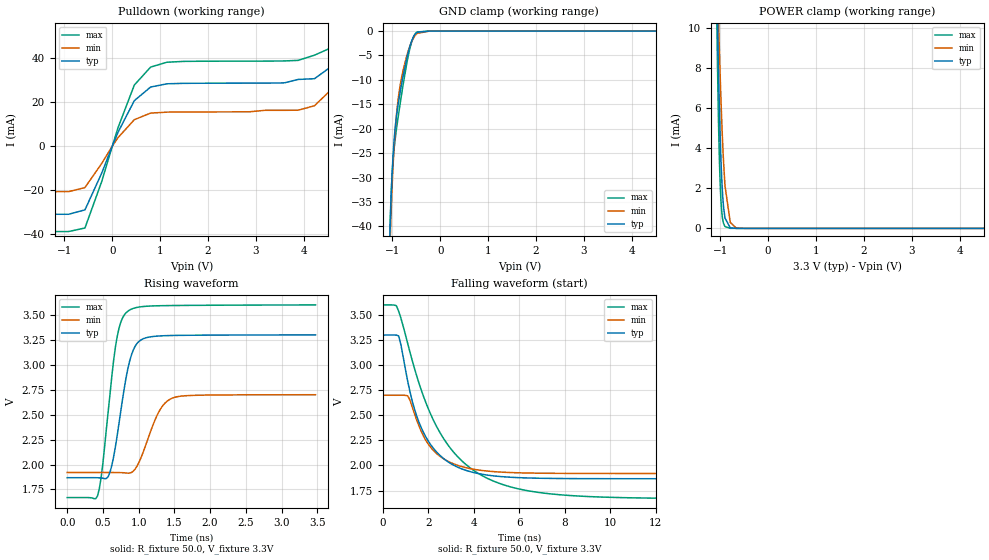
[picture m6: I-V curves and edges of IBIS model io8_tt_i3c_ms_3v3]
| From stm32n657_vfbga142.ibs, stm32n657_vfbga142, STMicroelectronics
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[Model]   io8_tt_i3c_ms_3v3
Model_type I/O_open_drain
Polarity   Non-Inverting
Enable   Active-Low
| CAP_THRESHOLD on pad IOTT is "UDTCAPC" :
| Rising=30.0% of vddiov33m   Falling=70.0% of vddiov33m
| C_comp min and max val. don't necessarily correlate with the min and max pvt
| but are the smallest and greatest pad capacitance found.
| var   typ   min   max
C_comp   1.30270pF  1.06445pF  2.26730pF
|C_comp_pulldown   1.30270pF  1.06445pF  2.26730pF
Vinl = 1.35V
Vinh = 1.8V
Vmeas = 1.65V   | Reference voltage for timing measurements
Cref  = 50.0pF   | Timing specification test load capacitance value
Rref  = 1.0MOhm   | Timing specification test load resistance value
Vref  = 1.815V   | Timing specification test load voltage
[Model Spec]
| TIME_THRESHOLD on pin ZIV08M is "CMOS" :
| Rising=50.0% of vddv08m   Falling=50.0% of vddv08m
Vinl 1.08570V 868.70000mV 1.21270V
Vinh 1.55630V 1.26330V 1.71030V
| variable   typ   min   max
[Temperature Range] 25.0 125.0 -40.0
| variable   typ   min   max
[Voltage Range] 3.3V 2.7V 3.6V
| variable   typ   min   max
[POWER Clamp Reference] 3.3V 2.7V 3.6V
| variable   typ   min   max
[GND Clamp Reference] 0V 0V 0V
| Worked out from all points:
|   slope of the pulldown table from 0 to 0.495 V, typ, clamps not added: 23.2 ohm
|   GND clamp passes 1 mA (typ) near -0.55 V on its own axis
|   POWER clamp passes 1 mA (typ) near -0.93 V on its own axis
|   rising waveform, R_fixture 50.0, V_fixture 3.3V: 20-80 % time 197ps typ, 258ps min, 178ps max; typ from 1.87 V to 3.3 V
|   falling waveform, R_fixture 50.0, V_fixture 3.3V: 20-80 % time 1.34ns typ, 1.26ns min, 2.34ns max; typ from 3.3 V to 1.87 V
[POWER Clamp]
-3.3V     1.353A     318.4mA    2.015A
-1.07V    12.07mA    13.62mA    10.38mA
-1.06V    10.79mA    12.67mA    8.742mA
-1.05V    9.57mA     11.75mA    7.25mA
-1.03V    7.34mA     9.996mA    4.745mA
-1V       4.587mA    7.593mA    2.212mA
-980mV    3.182mA    6.169mA    1.235mA
-950mV    1.703mA    4.334mA    479uA
-900mV    514.6uA    2.139mA    90.78uA
-790mV    28.73uA    299.8uA    2.713uA
-670mV    1.278uA    27.48uA    388.8nA
6.6V      0A         0A         0A
[GND Clamp]
-3.3V     -3.772A    -3.743A    -3.788A
-1.05V    -42.34mA   -45.44mA   -41.2mA
-1.04V    -38.9mA    -42mA      -37.88mA
-1.03V    -35.84mA   -38.88mA   -35.06mA
-1V       -28.57mA   -31.07mA   -28.88mA
-970mV    -23.48mA   -25.09mA   -24.97mA
-920mV    -18.07mA   -17.99mA   -20.63mA
-860mV    -13.91mA   -12.68mA   -16.46mA
-770mV    -9.031mA   -7.879mA   -10.78mA
-640mV    -3.394mA   -3.285mA   -3.897mA
-480mV    -254.3uA   -469.3uA   -191.8uA
6.6V      220.4nA    5.137uA    223.2nA
| variable   typ   min   max
[Pullup Reference] 3.3V 2.7V 3.6V
| variable   typ   min   max
[Pulldown Reference] 0V 0V 0V
[Pulldown]
-3.3V     -30.95mA   -20.65mA   -38.82mA
-570mV    -28.95mA   -18.8mA    -37.2mA
-220mV    -12.23mA   -7.828mA   -16.04mA
120mV     6.335mA    3.893mA    8.43mA
460mV     20.73mA    12.07mA    27.81mA
800mV     26.92mA    15.05mA    35.98mA
3.88V     30.37mA    16.38mA    39.04mA
4.22V     30.7mA     18.4mA     41.4mA
4.56V     36.08mA    25.54mA    44.69mA
4.9V      54.47mA    48.35mA    60.15mA
5.24V     110.5mA    112.9mA    109.4mA
6.6V      684.6mA    689.2mA    626.6mA
[Ramp]
dV/dt_r 858.15249mV/196.48606ps 467.16139mV/257.53913ps 1.15741V/176.93699ps
dV/dt_f 859.27463mV/1.33556ns 467.96319mV/1.25839ns 1.15858V/2.3342ns
R_load = 50.0
| Removed startup time: 0s 0s 0s  .
| Removed end time: 3.475ns.
[Rising Waveform]
R_fixture   = 50.0
V_fixture   = 3.3V
V_fixture_min = 2.7V
V_fixture_max = 3.6V
0s        1.868V     1.92V      1.669V
425ps     1.867V     1.92V      1.687V
475ps     1.865V     1.92V      1.87V
575ps     1.881V     1.92V      2.539V
675ps     2.179V     1.92V      3.176V
850ps     2.963V     1.913V     3.536V
1.025ns   3.244V     2.055V     3.579V
1.275ns   3.287V     2.517V     3.59V
1.475ns   3.292V     2.666V     3.592V
3.475ns   3.298V     2.699V     3.598V
| Removed startup time: 0s 0s 0s  .
| Removed end time: 24.9ns.
[Falling Waveform]
R_fixture   = 50.0
V_fixture   = 3.3V
V_fixture_min = 2.7V
V_fixture_max = 3.6V
0s        3.3V       2.7V       3.6V
700ps     3.292V     2.7V       3.538V
1.1ns     2.838V     2.694V     3.215V
1.4ns     2.56V      2.513V     2.965V
1.8ns     2.325V     2.289V     2.684V
2.3ns     2.152V     2.133V     2.419V
3.5ns     1.964V     1.987V     2.041V
5.2ns     1.889V     1.934V     1.816V
9.9ns     1.868V     1.92V      1.683V
24.9ns    1.868V     1.92V      1.669V
